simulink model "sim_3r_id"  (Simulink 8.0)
settings: Solver=ode45  StartTime=0.0  StopTime=5  RelTol=1e-3  AbsTol=1e-3
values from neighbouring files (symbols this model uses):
  m = 1    [mechanical_system.m]
  s = Lv/norm(Lv)    [pkm1.m]
undefined symbols (not defined in the file or in its folder): deg, kg, mN, N, rad
libraries: mblibv1 x18

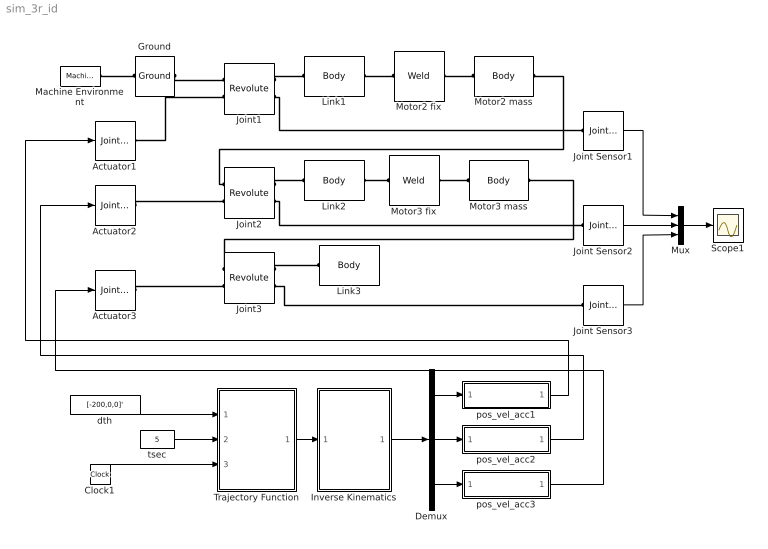
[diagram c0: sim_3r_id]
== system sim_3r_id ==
  Actuator1 : mblibv1/Sensors &  Actuators/Joint Actuator  UpdateFromCAD=off  PhysicalDomain=Mechanical  PortType=blob  ActuationStyle=Motion  AngleUnits=rad  ArcVelocityUnits=rad/s  ArcAccelerationUnits=rad/s^2  CoordPositionUnits=m  VelocityUnits=m/s  AccelerationUnits=m/s^2  ForceUnits=N  TorqueUnits=N*m  ActiveIO=on  Width=3  DialogClass=MechanicalActuatorBlock  Primitive=R1  ReferenceFrame=Absolute (World)
  Actuator2 : mblibv1/Sensors &  Actuators/Joint Actuator  UpdateFromCAD=off  PhysicalDomain=Mechanical  PortType=blob  ActuationStyle=Motion  AngleUnits=rad  ArcVelocityUnits=rad/s  ArcAccelerationUnits=rad/s^2  CoordPositionUnits=m  VelocityUnits=m/s  AccelerationUnits=m/s^2  ForceUnits=N  TorqueUnits=N*m  ActiveIO=on  Width=3  DialogClass=MechanicalActuatorBlock  Primitive=R1  ReferenceFrame=Absolute (World)
  Actuator3 : mblibv1/Sensors &  Actuators/Joint Actuator  UpdateFromCAD=off  PhysicalDomain=Mechanical  PortType=blob  ActuationStyle=Motion  AngleUnits=rad  ArcVelocityUnits=rad/s  ArcAccelerationUnits=rad/s^2  CoordPositionUnits=m  VelocityUnits=m/s  AccelerationUnits=m/s^2  ForceUnits=N  TorqueUnits=N*m  ActiveIO=on  Width=3  DialogClass=MechanicalActuatorBlock  Primitive=R1  ReferenceFrame=Absolute (World)
  Clock1 : Clock
  Demux : Demux  Outputs=3
  Ground : mblibv1/Bodies/Ground  UpdateFromCAD=off  LeftPortType=env  RightPortType=workingframe  PhysicalDomain=Mechanical  DialogClass=GroundBlock  CoordPosition=[0 0 0]  CoordPositionUnits=m  StateVectorMgrId=4  MachineId=[5 0]  ShowEnvPort=on
  Inverse Kinematics : MATLAB Function  TreatAsAtomicUnit=on
  Joint Sensor1 : mblibv1/Sensors &  Actuators/Joint Sensor  UpdateFromCAD=off  PhysicalDomain=Mechanical  PortType=blob  Muxed=on  Pose=off  Angle=off  AngleUnits=deg  ArcVelocity=off  ArcVelocityUnits=deg/s  ArcAcceleration=off  ArcAccelerationUnits=deg/s^2  CoordPosition=on  CoordPositionUnits=m  Velocity=off  VelocityUnits=m/s  Acceleration=off  AccelerationUnits=m/s^2  Quaternion=on  QuaternionDT=off  QuaternionDDT=off  QuaternionUnits=off  OutputVector=[1]  ActiveIO=on  Width=1  DialogClass=MechanicalSensorBlock  Primitive=R1  Force=off  ForceUnits=N  Torque=on  TorqueUnits=mN*m  ReferenceFrame=Absolute (World)  ReactionSensedSide=Base  ReactionReferenceFrame=Absolute (World)  ReactionForce=off  ReactionForceUnits=N  ReactionMoment=off  ReactionMomentUnits=N*m
  Joint Sensor2 : mblibv1/Sensors &  Actuators/Joint Sensor  UpdateFromCAD=off  PhysicalDomain=Mechanical  PortType=blob  Muxed=on  Pose=off  Angle=off  AngleUnits=deg  ArcVelocity=off  ArcVelocityUnits=deg/s  ArcAcceleration=off  ArcAccelerationUnits=deg/s^2  CoordPosition=on  CoordPositionUnits=m  Velocity=off  VelocityUnits=m/s  Acceleration=off  AccelerationUnits=m/s^2  Quaternion=on  QuaternionDT=off  QuaternionDDT=off  QuaternionUnits=off  OutputVector=[1]  ActiveIO=on  Width=1  DialogClass=MechanicalSensorBlock  Primitive=R1  Force=off  ForceUnits=N  Torque=on  TorqueUnits=mN*m  ReferenceFrame=Absolute (World)  ReactionSensedSide=Base  ReactionReferenceFrame=Absolute (World)  ReactionForce=off  ReactionForceUnits=N  ReactionMoment=off  ReactionMomentUnits=N*m
  Joint Sensor3 : mblibv1/Sensors &  Actuators/Joint Sensor  UpdateFromCAD=off  PhysicalDomain=Mechanical  PortType=blob  Muxed=on  Pose=off  Angle=off  AngleUnits=deg  ArcVelocity=off  ArcVelocityUnits=deg/s  ArcAcceleration=off  ArcAccelerationUnits=deg/s^2  CoordPosition=on  CoordPositionUnits=m  Velocity=off  VelocityUnits=m/s  Acceleration=off  AccelerationUnits=m/s^2  Quaternion=on  QuaternionDT=off  QuaternionDDT=off  QuaternionUnits=off  OutputVector=[1]  ActiveIO=on  Width=1  DialogClass=MechanicalSensorBlock  Primitive=R1  Force=off  ForceUnits=N  Torque=on  TorqueUnits=mN*m  ReferenceFrame=Absolute (World)  ReactionSensedSide=Base  ReactionReferenceFrame=Absolute (World)  ReactionForce=off  ReactionForceUnits=N  ReactionMoment=off  ReactionMomentUnits=N*m
  Joint1 : mblibv1/Joints/Revolute  LConnTagsString=__newl0|SA1  RConnTagsString=__newr0|SA1  UpdateFromCAD=off  NumSAPorts=2  CutJoint=off  MarkAsCut=off  Primitives=prismatic  PrimitiveProps=R1$World$[0 0 1]$revolute  DialogClass=JointBlock  R1Axis=[0 0 1]
  Joint2 : mblibv1/Joints/Revolute  LConnTagsString=__newl0|SA1  RConnTagsString=__newr0|SA1  UpdateFromCAD=off  NumSAPorts=2  CutJoint=off  MarkAsCut=off  Primitives=prismatic  PrimitiveProps=R1$World$[0 0 1]$revolute  DialogClass=JointBlock  R1Axis=[0 0 1]
  Joint3 : mblibv1/Joints/Revolute  LConnTagsString=__newl0|SA1  RConnTagsString=__newr0|SA1  UpdateFromCAD=off  NumSAPorts=2  CutJoint=off  MarkAsCut=off  Primitives=prismatic  PrimitiveProps=R1$World$[0 0 1]$revolute  DialogClass=JointBlock  R1Axis=[0 0 1]
  Link1 : mblibv1/Bodies/Body  LConnTagsString=CS1  RConnTagsString=CS2  UpdateFromCAD=off  DialogClass=MechanicalBodyBlock  Mass=0.071  MassUnits=kg  InertiaUnits=kg*m^2  Inertia=[0.000089395 0 0; 0 0.000089395 0; 0 0 0]  Shape=Cylinder  ShapeDims=[1 1]  ShapeUnits=m  ShapeUse=false  Density=1  DensityUnits=kg/m^3  DensityUse=false  GraphicsMode=MACHINE_DEFAULT  BodyColorSelMode=MACHINE_DEFAULT  BodyColor=[1 0 0]  AttachedToCS=CG  CG=Left$CG$[0.0373 0 0]$CS1$CS1$m$[0 0 0]$Euler X-Y-Z$deg$WORLD$false$none  WorkingFrames=Left$CS1$[0 0 0]$World$World$m$[0 0 0]$Euler X-Y-Z$deg$WORLD$true$none#Right$CS2$[0.1 0 0]$World$World$m$[0 0 0]$Euler X-Y-Z$deg$WORLD$true$none  CGPos=[0.0373 0 0]  CGRot=[0 0 0]  CS0Pos=[]  CS0Rot=[]  CS1Pos=[0 0 0]  CS1Rot=[0 0 0]  CS2Pos=[0.1 0 0]  CS2Rot=[0 0 0]  CS3Pos=[]  CS3Rot=[]  CS4Pos=[]  CS4Rot=[]  CS5Pos=[]  CS5Rot=[]  CS6Pos=[]  CS6Rot=[]  CS7Pos=[]  CS7Rot=[]  CS8Pos=[]  CS8Rot=[]  CS9Pos=[]  CS9Rot=[]  CS10Pos=[]  CS10Rot=[]  CS11Pos=[]  CS11Rot=[]  CS12Pos=[]  CS12Rot=[]  CS13Pos=[]  CS13Rot=[]  CS14Pos=[]  CS14Rot=[]  CS15Pos=[]  CS15Rot=[]  CS16Pos=[]  CS16Rot=[]  CS17Pos=[]  CS17Rot=[]  CS18Pos=[]  CS18Rot=[]  CS19Pos=[]  CS19Rot=[]  CS20Pos=[]  CS20Rot=[]
  Link2 : mblibv1/Bodies/Body  LConnTagsString=CS1  RConnTagsString=CS2  UpdateFromCAD=off  DialogClass=MechanicalBodyBlock  Mass=0.055  MassUnits=kg  InertiaUnits=kg*m^2  Inertia=[0.000038709 0 0; 0 0.000038709 0; 0 0 0]  Shape=Cylinder  ShapeDims=[1 1]  ShapeUnits=m  ShapeUse=false  Density=1  DensityUnits=kg/m^3  DensityUse=false  GraphicsMode=MACHINE_DEFAULT  BodyColorSelMode=MACHINE_DEFAULT  BodyColor=[1 0 0]  AttachedToCS=CG  CG=Left$CG$[0.0236 0 0]$CS1$CS1$m$[0 0 0]$Euler X-Y-Z$deg$WORLD$false$none  WorkingFrames=Left$CS1$[0.1 0 0]$World$World$m$[0 0 0]$Euler X-Y-Z$deg$WORLD$true$none#Right$CS2$[0.17 0 0]$World$World$m$[0 0 0]$Euler X-Y-Z$deg$WORLD$true$none  CGPos=[0.0236 0 0]  CGRot=[0 0 0]  CS0Pos=[]  CS0Rot=[]  CS1Pos=[0.1 0 0]  CS1Rot=[0 0 0]  CS2Pos=[0.17 0 0]  CS2Rot=[0 0 0]  CS3Pos=[]  CS3Rot=[]  CS4Pos=[]  CS4Rot=[]  CS5Pos=[]  CS5Rot=[]  CS6Pos=[]  CS6Rot=[]  CS7Pos=[]  CS7Rot=[]  CS8Pos=[]  CS8Rot=[]  CS9Pos=[]  CS9Rot=[]  CS10Pos=[]  CS10Rot=[]  CS11Pos=[]  CS11Rot=[]  CS12Pos=[]  CS12Rot=[]  CS13Pos=[]  CS13Rot=[]  CS14Pos=[]  CS14Rot=[]  CS15Pos=[]  CS15Rot=[]  CS16Pos=[]  CS16Rot=[]  CS17Pos=[]  CS17Rot=[]  CS18Pos=[]  CS18Rot=[]  CS19Pos=[]  CS19Rot=[]  CS20Pos=[]  CS20Rot=[]
  Link3 : mblibv1/Bodies/Body  LConnTagsString=CS1  UpdateFromCAD=off  DialogClass=MechanicalBodyBlock  Mass=0.05  MassUnits=kg  InertiaUnits=kg*m^2  Inertia=[0.000024587 0 0; 0 0.000024587 0; 0 0 0]  Shape=Cylinder  ShapeDims=[1 1]  ShapeUnits=m  ShapeUse=false  Density=1  DensityUnits=kg/m^3  DensityUse=false  GraphicsMode=MACHINE_DEFAULT  BodyColorSelMode=MACHINE_DEFAULT  BodyColor=[1 0 0]  AttachedToCS=CG  CG=Left$CG$[0.0186 0 0]$CS1$CS1$m$[0 0 0]$Euler X-Y-Z$deg$WORLD$false$none  WorkingFrames=Left$CS1$[0.17 0 0]$World$World$m$[0 0 0]$Euler X-Y-Z$deg$WORLD$true$none#Right$CS2$[0.22 0 0]$World$World$m$[0 0 0]$Euler X-Y-Z$deg$WORLD$false$none  CGPos=[0.0186 0 0]  CGRot=[0 0 0]  CS0Pos=[]  CS0Rot=[]  CS1Pos=[0.17 0 0]  CS1Rot=[0 0 0]  CS2Pos=[0.22 0 0]  CS2Rot=[0 0 0]  CS3Pos=[]  CS3Rot=[]  CS4Pos=[]  CS4Rot=[]  CS5Pos=[]  CS5Rot=[]  CS6Pos=[]  CS6Rot=[]  CS7Pos=[]  CS7Rot=[]  CS8Pos=[]  CS8Rot=[]  CS9Pos=[]  CS9Rot=[]  CS10Pos=[]  CS10Rot=[]  CS11Pos=[]  CS11Rot=[]  CS12Pos=[]  CS12Rot=[]  CS13Pos=[]  CS13Rot=[]  CS14Pos=[]  CS14Rot=[]  CS15Pos=[]  CS15Rot=[]  CS16Pos=[]  CS16Rot=[]  CS17Pos=[]  CS17Rot=[]  CS18Pos=[]  CS18Rot=[]  CS19Pos=[]  CS19Rot=[]  CS20Pos=[]  CS20Rot=[]
  Machine Environment : mblibv1/Bodies/Machine Environment  PortType=env  PhysicalDomain=Mechanical  DialogTemplateClass=MECH.MachineEnvironment  SyncWhenCopied=off  Gravity=[0 -9.81 0]  GravityUnits=m/s^2  GravityAsSignal=off  Dimensionality=Auto-detect  AnalysisType=Inverse dynamics  LinearAssemblyTolerance=1e-3  LinearAssemblyToleranceUnits=m  AngularAssemblyTolerance=1e-3  AngularAssemblyToleranceUnits=rad  ConstraintSolverType=Stabilizing  ConstraintRelTolerance=1e-4  ConstraintAbsTolerance=1e-4  UseRobustSingularityHandling=off  RedundancyAnalysisToleranceType=Automatically select tolerance  RedundancyAnalysisTolerance=1e-14  StatePerturbationType=Fixed  PerturbationSize=1e-5  VisualizeMachine=on  BodyVisualizationType=Use model default body geometries  BodyColorSelMode=Use model default  DefaultBodyColor=[1 0 0]
  Motor2 fix : mblibv1/Joints/Weld  LConnTagsString=__newl0  RConnTagsString=__newr0  UpdateFromCAD=off  NumSAPorts=0  CutJoint=off  MarkAsCut=off  Primitives=weld  PrimitiveProps=W$WORLD$[0 0 0]$weld  DialogClass=JointBlock  WAxis=[0 0 0]
  Motor2 mass : mblibv1/Bodies/Body  LConnTagsString=CS1  RConnTagsString=CS2  UpdateFromCAD=off  DialogClass=MechanicalBodyBlock  Mass=0.292  MassUnits=kg  InertiaUnits=kg*m^2  Inertia=[0 0 0; 0 0 0; 0 0 0]  Shape=Cylinder  ShapeDims=[1 1]  ShapeUnits=m  ShapeUse=false  Density=1  DensityUnits=kg/m^3  DensityUse=false  GraphicsMode=MACHINE_DEFAULT  BodyColorSelMode=MACHINE_DEFAULT  BodyColor=[1 0 0]  AttachedToCS=CG  CG=Left$CG$[0.1 0 0]$WORLD$WORLD$m$[0 0 0]$Euler X-Y-Z$deg$WORLD$false$none  WorkingFrames=Left$CS1$[0.1 0 0]$World$World$m$[0 0 0]$Euler X-Y-Z$deg$WORLD$true$none#Right$CS2$[0.1 0 0]$World$World$m$[0 0 0]$Euler X-Y-Z$deg$WORLD$true$none  CGPos=[0.1 0 0]  CGRot=[0 0 0]  CS0Pos=[]  CS0Rot=[]  CS1Pos=[0.1 0 0]  CS1Rot=[0 0 0]  CS2Pos=[0.1 0 0]  CS2Rot=[0 0 0]  CS3Pos=[]  CS3Rot=[]  CS4Pos=[]  CS4Rot=[]  CS5Pos=[]  CS5Rot=[]  CS6Pos=[]  CS6Rot=[]  CS7Pos=[]  CS7Rot=[]  CS8Pos=[]  CS8Rot=[]  CS9Pos=[]  CS9Rot=[]  CS10Pos=[]  CS10Rot=[]  CS11Pos=[]  CS11Rot=[]  CS12Pos=[]  CS12Rot=[]  CS13Pos=[]  CS13Rot=[]  CS14Pos=[]  CS14Rot=[]  CS15Pos=[]  CS15Rot=[]  CS16Pos=[]  CS16Rot=[]  CS17Pos=[]  CS17Rot=[]  CS18Pos=[]  CS18Rot=[]  CS19Pos=[]  CS19Rot=[]  CS20Pos=[]  CS20Rot=[]
  Motor3 fix : mblibv1/Joints/Weld  LConnTagsString=__newl0  RConnTagsString=__newr0  UpdateFromCAD=off  NumSAPorts=0  CutJoint=off  MarkAsCut=off  Primitives=weld  PrimitiveProps=W$WORLD$[0 0 0]$weld  DialogClass=JointBlock  WAxis=[0 0 0]
  Motor3 mass : mblibv1/Bodies/Body  LConnTagsString=CS1  RConnTagsString=CS2  UpdateFromCAD=off  DialogClass=MechanicalBodyBlock  Mass=0.292  MassUnits=kg  InertiaUnits=kg*m^2  Inertia=[0 0 0; 0 0 0; 0 0 0]  Shape=Cylinder  ShapeDims=[1 1]  ShapeUnits=m  ShapeUse=false  Density=1  DensityUnits=kg/m^3  DensityUse=false  GraphicsMode=MACHINE_DEFAULT  BodyColorSelMode=MACHINE_DEFAULT  BodyColor=[1 0 0]  AttachedToCS=CG  CG=Left$CG$[0.17 0 0]$WORLD$WORLD$m$[0 0 0]$Euler X-Y-Z$deg$WORLD$false$none  WorkingFrames=Left$CS1$[0.17 0 0]$World$World$m$[0 0 0]$Euler X-Y-Z$deg$WORLD$true$none#Right$CS2$[0.17 0 0]$World$World$m$[0 0 0]$Euler X-Y-Z$deg$WORLD$true$none  CGPos=[0.17 0 0]  CGRot=[0 0 0]  CS0Pos=[]  CS0Rot=[]  CS1Pos=[0.17 0 0]  CS1Rot=[0 0 0]  CS2Pos=[0.17 0 0]  CS2Rot=[0 0 0]  CS3Pos=[]  CS3Rot=[]  CS4Pos=[]  CS4Rot=[]  CS5Pos=[]  CS5Rot=[]  CS6Pos=[]  CS6Rot=[]  CS7Pos=[]  CS7Rot=[]  CS8Pos=[]  CS8Rot=[]  CS9Pos=[]  CS9Rot=[]  CS10Pos=[]  CS10Rot=[]  CS11Pos=[]  CS11Rot=[]  CS12Pos=[]  CS12Rot=[]  CS13Pos=[]  CS13Rot=[]  CS14Pos=[]  CS14Rot=[]  CS15Pos=[]  CS15Rot=[]  CS16Pos=[]  CS16Rot=[]  CS17Pos=[]  CS17Rot=[]  CS18Pos=[]  CS18Rot=[]  CS19Pos=[]  CS19Rot=[]  CS20Pos=[]  CS20Rot=[]
  Mux : Mux  Inputs=3
  Scope1 : Scope
  Trajectory Function : MATLAB Function  TreatAsAtomicUnit=on
  dth : Constant  Value=[-200,0,0]'  SampleTime=-1
  pos_vel_acc1 : Subsystem
  pos_vel_acc2 : Subsystem
  pos_vel_acc3 : Subsystem
  tsec : Constant  Value=5  SampleTime=-1
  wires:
  Clock1/1 -> Trajectory Function/3(tout)
  tsec/1 -> Trajectory Function/2(tsec)
  dth/1 -> Trajectory Function/1(dx)
  Inverse Kinematics/1(thd) -> Demux/1
  Trajectory Function/1(xd) -> Inverse Kinematics/1(xd)
  Joint Sensor1/1 -> Mux/1
  Joint Sensor2/1 -> Mux/2
  Joint Sensor3/1 -> Mux/3
  Mux/1 -> Scope1/1
  Demux/1 -> pos_vel_acc1/1(In1)
  Demux/2 -> pos_vel_acc2/1(In1)
  Demux/3 -> pos_vel_acc3/1(In1)
  pos_vel_acc1/1(Motion1) -> Actuator1/1
  pos_vel_acc2/1(Motion1) -> Actuator2/1
  pos_vel_acc3/1(Motion1) -> Actuator3/1
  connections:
  Ground/RConn1 -- Joint1/LConn1
  Joint1/RConn1 -- Link1/LConn1
  Machine Environment/RConn1 -- Ground/LConn1
  Motor2 fix/RConn1 -- Motor2 mass/LConn1
  Link1/RConn1 -- Motor2 fix/LConn1
  Joint2/RConn1 -- Link2/LConn1
  Joint3/RConn1 -- Link3/LConn1
  Motor3 fix/RConn1 -- Motor3 mass/LConn1
  Motor3 fix/LConn1 -- Link2/RConn1
  Joint2/LConn1 -- Motor2 mass/RConn1
  Joint3/LConn1 -- Motor3 mass/RConn1
  Actuator1/RConn1 -- Joint1/LConn2
  Joint1/RConn2 -- Joint Sensor1/LConn1
  Joint2/RConn2 -- Joint Sensor2/LConn1
  Joint3/RConn2 -- Joint Sensor3/LConn1
  Actuator2/RConn1 -- Joint2/LConn2
  Actuator3/RConn1 -- Joint3/LConn2

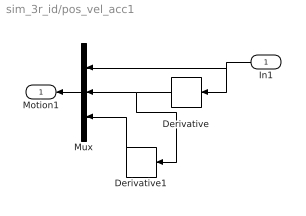
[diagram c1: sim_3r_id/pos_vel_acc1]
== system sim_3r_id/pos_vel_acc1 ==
  In1 : Inport
  Derivative : Derivative
  Derivative1 : Derivative
  Mux : Mux  Inputs=3
  Motion1 : Outport
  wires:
  Mux/1 -> Motion1/1
  Derivative/1 -> Mux/2, Derivative1/1
  Derivative1/1 -> Mux/3
  In1/1 -> Mux/1, Derivative/1

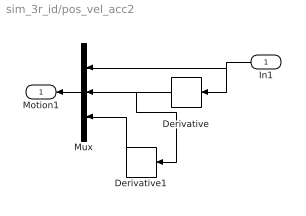
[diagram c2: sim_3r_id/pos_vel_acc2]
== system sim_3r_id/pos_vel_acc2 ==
  In1 : Inport
  Derivative : Derivative
  Derivative1 : Derivative
  Mux : Mux  Inputs=3
  Motion1 : Outport
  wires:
  Mux/1 -> Motion1/1
  Derivative/1 -> Mux/2, Derivative1/1
  Derivative1/1 -> Mux/3
  In1/1 -> Mux/1, Derivative/1

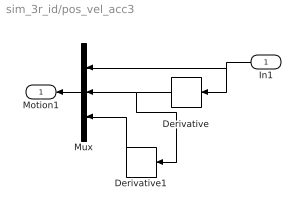
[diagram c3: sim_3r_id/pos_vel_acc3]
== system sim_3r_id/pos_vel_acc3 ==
  In1 : Inport
  Derivative : Derivative
  Derivative1 : Derivative
  Mux : Mux  Inputs=3
  Motion1 : Outport
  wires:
  Mux/1 -> Motion1/1
  Derivative/1 -> Mux/2, Derivative1/1
  Derivative1/1 -> Mux/3
  In1/1 -> Mux/1, Derivative/1

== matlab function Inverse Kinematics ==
function thd  = fcn(xd)

persistent index thd_p

% Initializing Variables %
if isempty(index), index=0; end
if isempty(thd_p), thd_p=(pi/180)*[0,90,0]'; end

w_index=1;  % In workspace %
a1=100; a2=70; a3=50;

qx=xd(1,1); qy=xd(2,1); phi=xd(3,1);

% (1) Calculate th2 %
px=qx-a3*cos(phi); py=qy-a3*sin(phi);
kapha=(px^2+py^2-a1^2-a2^2)/(2*a1*a2);
if abs(kapha)>1
    w_index=-1;  % Out of Workspace %
    kapha=1;
end
th2=+acos(kapha); % Elbow Down %
%th2=-acos(kapha); % Elbow Up %
 
% (2) Calculate th1 %
delta=a1^2+a2^2+2*a1*a2*cos(th2);
cth1=(px*(a1+a2*cos(th2))+py*a2*sin(th2))/delta;
sth1=(-px*a2*sin(th2)+py*(a1+a2*cos(th2)))/delta;
th1=atan2(sth1, cth1);
if th1<0, th1=th1+2*pi; end % 0<th<360 %

% (3) Calcuate th3 %
th3=phi-(th1+th2);

% (3) Check Joint Limits %
if th1<0 || th1>pi, w_index=-1; end
if th2<pi/6 || th2>5*pi/6, w_index=-1; end

% Result %
if w_index==1
    thd=[th1, th2, th3]';
else
    thd=thd_p;
end

% Save the current value %
thd_p=thd;

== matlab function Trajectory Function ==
function xd = fcn(dx, tsec, tout)

MAX_CH=3;       % Two Actuators %
a1=100; a2=70; a3=50;

% Initializing Variables %
xd=zeros(MAX_CH,1);
x0=[a1,a2+a3, pi/2]';

%tout=index*dt;

    [c] = coeff_3rd(x0, zeros(MAX_CH,1), x0+dx, zeros(MAX_CH,1), tsec);
    for ch=1:MAX_CH
        xd(ch,1)=c(ch,1)+c(ch,2)*tout+c(ch,3)*tout^2+c(ch,4)*tout^3;    
    end

function [c] = coeff_3rd(sp, sv, ep, ev, tsec)
MAX_CH=3;
c=zeros(MAX_CH,4);
for ch=1:MAX_CH
    c(ch,1)=sp(ch,1);
    c(ch,2)=sv(ch,1);
    c(ch,3)=(3.0*(ep(ch,1)-sp(ch,1))-(2.0*sv(ch,1)+ev(ch,1))*tsec)/(tsec*tsec);
    c(ch,4)=(-2.0*(ep(ch,1)-sp(ch,1))+(sv(ch,1)+ev(ch,1))*tsec)/(tsec*tsec*tsec);
end
